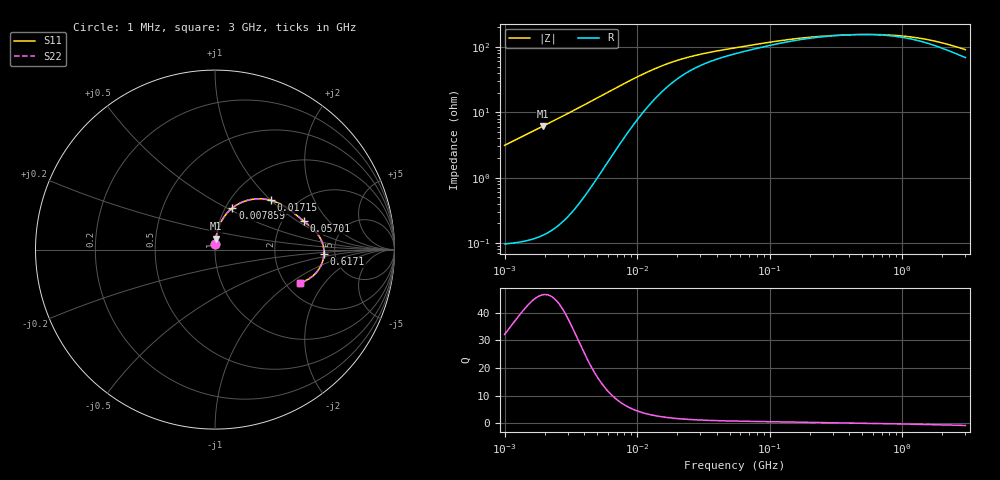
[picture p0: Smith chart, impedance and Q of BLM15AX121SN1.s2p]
! BLM15AX121SN1
# Hz S RI R 50
!Freq.(Hz) S11(Real) S11(Imag) S21(Real) S21(Imag) S12(Real) S12(Imag) S22(Real) S22(Imag)
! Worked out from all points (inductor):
!   401 points, 1 MHz to 3 GHz, reference 50 ohm
!   read as one part in series: L = 497 nH near 1.041 MHz
!   highest Q = 46.6 at 1.936 MHz (marker M1), where L = 501 nH
!   self-resonance near 461.7 MHz
!   S11 on the Smith chart (normalised r, x): 1 MHz: 1.00, +0.06; 7.859 MHz: 1.08, +0.53; 17.15 MHz: 1.50, +1.00; 57.01 MHz: 2.60, +1.13; 617.1 MHz: 4.07, -0.33; 3 GHz: 2.37, -1.19
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1000000  0.00194 0.0311  0.9981 -0.0311  0.9981 -0.0311  0.00194 0.0311
1935809  0.00499 0.0605  0.995 -0.0605  0.995 -0.0605  0.00499 0.0605
2775447  0.00985 0.0873  0.9902 -0.0873  0.9902 -0.0873  0.00985 0.0873
3823119  0.0194 0.1209  0.9806 -0.1209  0.9806 -0.1209  0.0194 0.1209
5705239  0.048 0.1786  0.952 -0.1786  0.952 -0.1786  0.048 0.1786
7858845  0.0972 0.2321  0.9028 -0.2321  0.9028 -0.2321  0.0972 0.2321
1.082539e7  0.1766 0.2734  0.8234 -0.2734  0.8234 -0.2734  0.1766 0.2734
1.461624e7  0.2653 0.2823  0.7347 -0.2823  0.7347 -0.2823  0.2653 0.2823
1.71545e7  0.3101 0.2745  0.6899 -0.2745  0.6899 -0.2745  0.3101 0.2745
2.181181e7  0.3672 0.2524  0.6328 -0.2524  0.6328 -0.2524  0.3672 0.2524
2.829425e7  0.4142 0.2233  0.5858 -0.2233  0.5858 -0.2233  0.4142 0.2233
5.477226e7  0.4907 0.1615  0.5093 -0.1615  0.5093 -0.1615  0.4907 0.1615
5.700937e7  0.4945 0.1585  0.5055 -0.1585  0.5055 -0.1585  0.4945 0.1585
1.171891e8  0.5551 0.1066  0.4449 -0.1066  0.4449 -0.1066  0.5551 0.1066
2.094008e8  0.5874 0.0617  0.4126 -0.0617  0.4126 -0.0617  0.5874 0.0617
3.667557e8  0.6036 0.0186  0.3964 -0.0186  0.3964 -0.0186  0.6036 0.0186
6.171487e8  0.6075 -0.0253  0.3925 0.0253  0.3925 0.0253  0.6075 -0.0253
8.005644e8  0.604 -0.0502  0.396 0.0502  0.396 0.0502  0.604 -0.0502
1.125055e9  0.5915 -0.0866  0.4085 0.0866  0.4085 0.0866  0.5915 -0.0866
1.581072e9  0.5661 -0.1258  0.4339 0.1258  0.4339 0.1258  0.5661 -0.1258
2.092429e9  0.5325 -0.1567  0.4675 0.1567  0.4675 0.1567  0.5325 -0.1567
3e9  0.4723 -0.1854  0.5277 0.1854  0.5277 0.1854  0.4723 -0.1854
